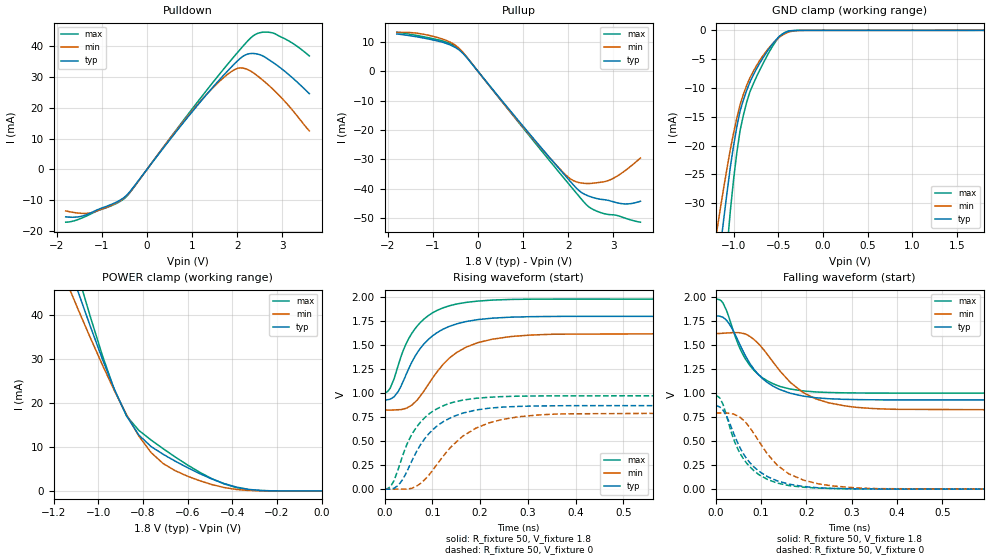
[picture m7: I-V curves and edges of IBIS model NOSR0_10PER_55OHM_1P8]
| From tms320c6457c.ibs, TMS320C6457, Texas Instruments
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|   Model Cell NOSR0_10PER_55OHM_1P8
|NOSR0_10PER_55OHM_1P8
[Model]   NOSR0_10PER_55OHM_1P8
Model_type   3-state
Polarity   Non-Inverting
Enable   Active-Low
Cref =  15.0000pF
Rref =  100.0000M
Vref =  0V
Vmeas =  0.9
C_comp   1.89p   1.72p   2.18p
[Model Spec]
Rref 50 NA NA
Vref 0.9 0.81 0.99
[Temperature Range]   25   125   -40
[Voltage Range]   1.8   1.62   1.98
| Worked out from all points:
|   slope of the pulldown table from 0 to 0.27 V, typ, clamps not added: 52.3 ohm
|   slope of the pullup table from 0 to 0.27 V, typ, clamps not added: 52.9 ohm
|   GND clamp passes 1 mA (typ) near -0.48 V on its own axis
|   POWER clamp passes 1 mA (typ) near -0.39 V on its own axis
|   rising waveform, R_fixture 50, V_fixture 1.8: 20-80 % time 71.3ps typ, 87.4ps min, 62.7ps max; typ from 0.929 V to 1.8 V
|   rising waveform, R_fixture 50, V_fixture 0: 20-80 % time 75.3ps typ, 95.9ps min, 64.2ps max; typ from 0 V to 0.871 V
|   falling waveform, R_fixture 50, V_fixture 1.8: 20-80 % time 75ps typ, 97.8ps min, 64.1ps max; typ from 1.8 V to 0.93 V
|   falling waveform, R_fixture 50, V_fixture 0: 20-80 % time 69.3ps typ, 85.4ps min, 60.8ps max; typ from 0.872 V to 0.001 V
| Nom Voltages:
|   BIAS2=0.9, BIASFET=0, VDD=1.1, VDDS=1.8, BUS_BIAS1=0, BUS_BIAS3=0,
|   VSS=0, VSSS=0
| Min Voltages:
|   BIAS2=0.81, BIASFET=0, VDD=0.99, VDDS=1.62, BUS_BIAS1=0, BUS_BIAS3=0,
|   VSS=0, VSSS=0
| Max Voltages:
|   BIAS2=0.99, BIASFET=0, VDD=1.21, VDDS=1.98, BUS_BIAS1=0, BUS_BIAS3=0,
|   VSS=0, VSSS=0
[POWER_clamp]
|   voltage   I(typ)   I(min)   I(max)
-1.8V     156mA      133.5mA    181.7mA
-1.127V   50.87mA    45.88mA    55.74mA
-1.109V   48.19mA    43.68mA    52.51mA
-1.073V   42.88mA    39.33mA    46.15mA
-1.055V   40.27mA    37.18mA    43.01mA
-927.3mV  23.11mA    22.83mA    22.99mA
-872.7mV  17.08mA    17.31mA    17.08mA
-818.2mV  12.73mA    12.5mA     13.8mA
-763.6mV  10.13mA    8.758mA    11.61mA
-600mV    5.297mA    3.359mA    5.911mA
-381.8mV  881.1uA    334.9uA    769uA
0V        130.3nA    147.3nA    381.2nA
[Pulldown]
|   voltage   I(typ)   I(min)   I(max)
-1.8V     -15.34mA   -13.43mA   -17.08mA
-1.527V   -15.36mA   -14.11mA   -16.22mA
-1.255V   -14.13mA   -14.06mA   -14.5mA
-490.9mV  -8.889mA   -9.054mA   -9.31mA
1.2V      22.17mA    22.36mA    23.35mA
1.691V    30.39mA    29.65mA    32.36mA
2.018V    35.33mA    32.8mA     38.08mA
2.291V    37.56mA    31.95mA    42.49mA
2.455V    37.38mA    30.27mA    44.1mA
2.673V    35.87mA    27.61mA    44.49mA
3.164V    30.48mA    20.28mA    41.48mA
3.6V      24.54mA    12.5mA     36.79mA
[Pullup]
|   voltage   I(typ)   I(min)   I(max)
-1.8V     12.78mA    13.28mA    13.41mA
-1.364V   11.81mA    13.05mA    12.28mA
-927.3mV  10.47mA    11.69mA    10.92mA
-600mV    8.904mA    9.83mA     9.357mA
-381.8mV  6.827mA    7.297mA    7.143mA
1.309V    -24.38mA   -24.61mA   -25.24mA
1.909V    -35.16mA   -34.81mA   -36.53mA
2.127V    -38.97mA   -37.38mA   -40.58mA
2.455V    -42.56mA   -38.27mA   -46.22mA
2.891V    -44.04mA   -37.24mA   -48.85mA
3.273V    -45.24mA   -33.72mA   -50.15mA
3.6V      -44.32mA   -29.56mA   -51.46mA
[GND_clamp]
|   voltage   I(typ)   I(min)   I(max)
-1.8V     -137.1mA   -107.1mA   -189.7mA
-1.182V   -42.18mA   -34.28mA   -58.62mA
-1.109V   -32.61mA   -27.18mA   -44.51mA
-1.073V   -28.08mA   -23.86mA   -37.8mA
-1.036V   -23.72mA   -20.65mA   -31.33mA
-963.6mV  -16.74mA   -15.21mA   -21.21mA
-927.3mV  -13.99mA   -12.88mA   -17.38mA
-854.5mV  -10.47mA   -9.599mA   -12.54mA
-781.8mV  -7.837mA   -7.198mA   -9.373mA
-600mV    -3.116mA   -2.961mA   -3.703mA
-418.2mV  -354.7uA   -522.3uA   -297.6uA
1.8V      130.3nA    2.912uA    201.9nA
[Ramp]
| variable   typ   min   max
dV/dt_f 0.43741558/58.801034p 0.40229927/76.089893p 0.49092051/50.17038p
dV/dt_r 0.43730293/58.957989p  0.3989897/75.364056p 0.48819124/50.510133p
R_load = 50
[Rising Waveform]
R_fixture = 50
V_fixture = 1.8
V_fixture_min = 1.62
V_fixture_max = 1.98
|   time   V(typ)   V(min)   V(max)
0s        928.7mV    825.8mV    1V
11.52ps   937.5mV    823.4mV    1.051V
28.55ps   1.018V     827.5mV    1.292V
46.24ps   1.208V     844.4mV    1.528V
68.35ps   1.422V     929.9mV    1.7V
100.1ps   1.597V     1.156V     1.836V
151.2ps   1.723V     1.425V     1.93V
225.2ps   1.781V     1.562V     1.97V
307.7ps   1.797V     1.606V     1.979V
1.185ns   1.8V       1.62V      1.98V
[Rising Waveform]
R_fixture = 50
V_fixture = 0
V_fixture_min = 0
V_fixture_max = 0
|   time   V(typ)   V(min)   V(max)
0s        0V         451.3uV    813.9uV
12.44ps   1.449mV    0V         27.89mV
28.55ps   39.16mV    0V         209.7mV
48.45ps   203.4mV    1.869mV    486.1mV
74.55ps   458.7mV    57.06mV    695.4mV
109.9ps   659.1mV    259.2mV    838.3mV
163.7ps   792.6mV    552.6mV    928mV
218.1ps   843.2mV    690.1mV    957.3mV
330.6ps   867.5mV    775.9mV    971.2mV
1.185ns   870.7mV    792.1mV    973.8mV
[Falling Waveform]
R_fixture = 50
V_fixture = 1.8
V_fixture_min = 1.62
V_fixture_max = 1.98
|   time   V(typ)   V(min)   V(max)
0s        1.8V       1.619V     1.98V
15.95ps   1.79V      1.624V     1.938V
29.95ps   1.721V     1.628V     1.778V
51.05ps   1.528V     1.63V      1.491V
74.85ps   1.313V     1.593V     1.291V
114ps     1.11V      1.403V     1.128V
164.5ps   999.2mV    1.112V     1.043V
220.9ps   952.1mV    940.4mV    1.013V
347.8ps   931.1mV    839.8mV    1.001V
1.185ns   929.9mV    826mV      1V
[Falling Waveform]
R_fixture = 50
V_fixture = 0
V_fixture_min = 0
V_fixture_max = 0
|   time   V(typ)   V(min)   V(max)
0s        872.4mV    793.7mV    974.9mV
9.648ps   852.9mV    793.7mV    944mV
22.95ps   770.2mV    792.3mV    780.8mV
44.55ps   524.5mV    771.4mV    461.6mV
68.35ps   317.6mV    683mV      270mV
114.4ps   130.5mV    364.7mV    101.3mV
161.6ps   52.82mV    159.1mV    38.06mV
225.9ps   15.04mV    56.58mV    11.99mV
322ps     3.48mV     11.26mV    3.674mV
1.185ns   1.008mV    877.6uV    625.7uV
